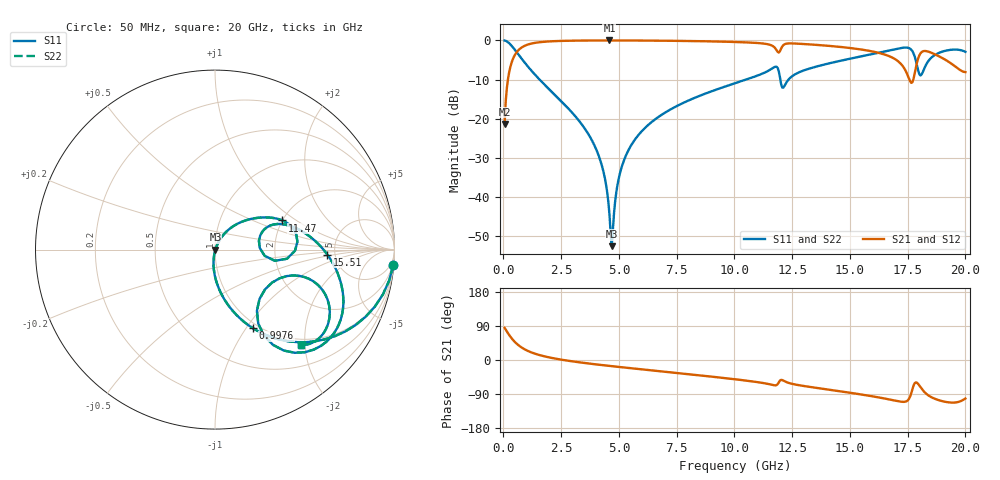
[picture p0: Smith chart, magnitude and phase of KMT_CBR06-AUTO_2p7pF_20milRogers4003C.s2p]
! Data measured by Modelithics Inc. support@modelithics.com 813-866-6335
! KEMET CBR06-AUTO 2.7pF, Pad Width= 0.851mm, Pad Length= 0.64mm, Pad Gap= 0.62mm, 20mil Rogers 4003C substrate Data, January 2022
# hz S ma R 50
! 2 Port Network Data from SP1.SP block
! freq  magS11  angS11  magS21  angS21  magS12  angS12  magS22  angS22
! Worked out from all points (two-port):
!   401 points, 50 MHz to 20 GHz, reference 50 ohm
!   highest |S21| = -0.02 dB at 4.589 GHz (marker M1); lowest = -21.3 dB at 50 MHz (marker M2)
!   |S21| within 3 dB of the highest: 574.2 MHz to 11.9 GHz (11.32 GHz wide, 182 % of centre); 11.93 GHz to 16.13 GHz (4.193 GHz wide, 29.9 % of centre)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
!   lowest |S11| = -52.6 dB at 4.688 GHz (marker M3), VSWR 1.00, Z = 50.2 - j0.0515 ohm
!   |S11| at or under -10 dB: 1.562 GHz to 10.51 GHz (8.951 GHz wide, 148 % of centre); 11.99 GHz to 12.35 GHz (358.6 MHz wide, 2.95 % of centre)
!   |S22| runs from -52.6 to 0.0 dB; largest |S21 - S12| = 0
!   S11 on the Smith chart (normalised r, x): 50 MHz: 1, -22; 997.6 MHz: 0.94, -1.08; 11.47 GHz: 2.00, +0.78; 15.51 GHz: 4.32, -0.40; 20 GHz: 0.88, -1.92
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5e7  0.9963 -5.1  0.08565 84.9  0.08565 84.9  0.9963 -5.1
3.4925e8  0.8557 -32.3  0.5164 57.6  0.5164 57.6  0.8557 -32.3
9.97625e8  0.4871 -64.2  0.872 25.7  0.872 25.7  0.4871 -64.2
3.391625e9  0.08446 -95.6  0.9943 -7.0  0.9943 -7.0  0.08446 -95.6
4.2395e9  0.02648 -98.4  0.9973 -13.2  0.9973 -13.2  0.02648 -98.4
4.588625e9  0.006033 -83.0  0.9975 -15.6  0.9975 -15.6  0.006033 -83.0
4.688375e9  0.002351 -12.6  0.9975 -16.3  0.9975 -16.3  0.002351 -12.6
4.987625e9  0.01701 63.5  0.9973 -18.3  0.9973 -18.3  0.01701 63.5
5.286875e9  0.03301 65.4  0.9968 -20.2  0.9968 -20.2  0.03301 65.4
6.73325e9  0.1063 59.0  0.9911 -29.4  0.9911 -29.4  0.1063 59.0
1.0025e10  0.2834 38.1  0.9536 -50.8  0.9536 -50.8  0.2834 38.1
1.147138e10  0.4093 23.4  0.8889 -63.3  0.8889 -63.3  0.4093 23.4
1.18205e10  0.4611 5.5  0.7542 -66.3  0.7542 -66.3  0.4611 5.5
1.211975e10  0.2494 11.1  0.8701 -54.4  0.8701 -54.4  0.2494 11.1
1.336662e10  0.447 16.7  0.8838 -71.9  0.8838 -71.9  0.447 16.7
1.551125e10  0.6269 -2.6  0.7628 -91.2  0.7628 -91.2  0.6269 -2.6
1.670825e10  0.7432 -17.4  0.6269 -104.1  0.6269 -104.1  0.7432 -17.4
1.765588e10  0.7603 -48.7  0.2865 -87.7  0.2865 -87.7  0.7603 -48.7
1.795512e10  0.4132 -55.6  0.5883 -63.2  0.5883 -63.2  0.4132 -55.6
1.825438e10  0.4604 -18.2  0.7319 -86.3  0.7319 -86.3  0.4604 -18.2
1.8803e10  0.6817 -23.6  0.6376 -105.2  0.6376 -105.2  0.6817 -23.6
2e10  0.7144 -48.0  0.3935 -101.6  0.3935 -101.6  0.7144 -48.0
